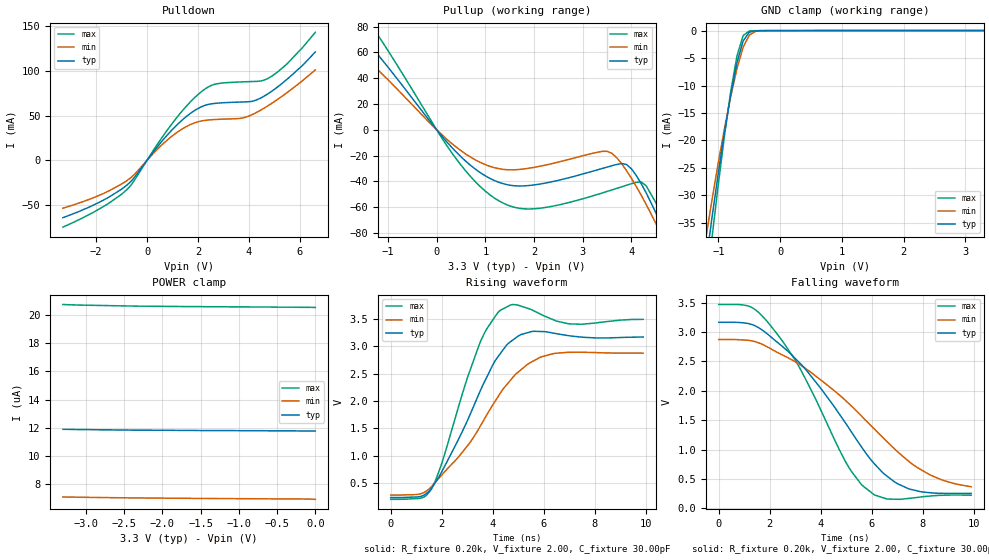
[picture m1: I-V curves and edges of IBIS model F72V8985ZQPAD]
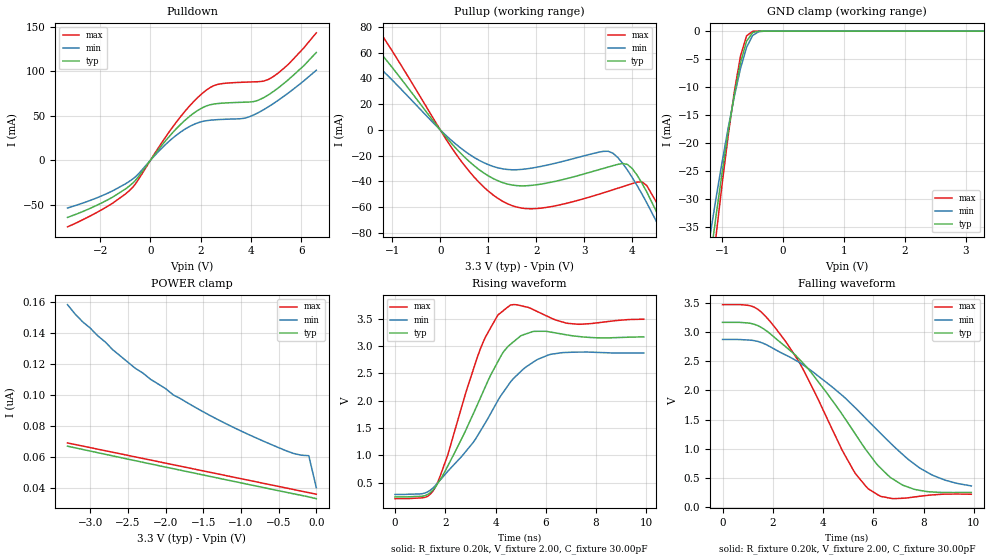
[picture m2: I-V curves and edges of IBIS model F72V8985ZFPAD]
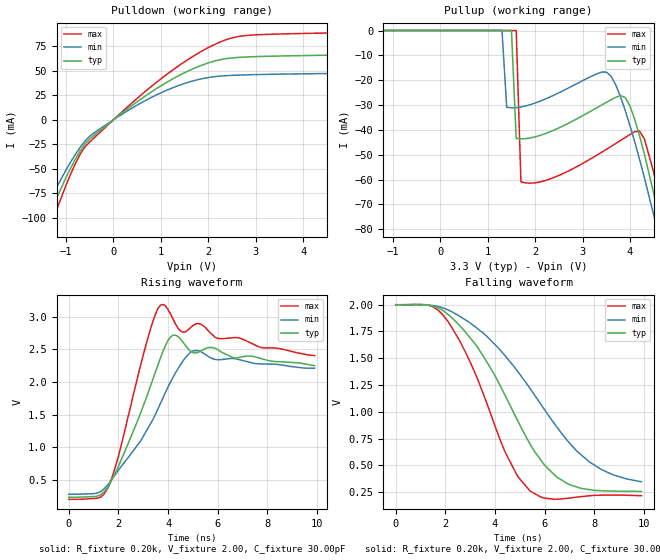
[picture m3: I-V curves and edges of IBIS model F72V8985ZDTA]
| IBIS file f72v8985.ibs created by s2ibis2 version 1.1
| North Carolina State University Electronics Research Laboratory  1995
[IBIS ver]   2.1
[File name]   f72v8985.ibs
[File Rev]   1.0
[Date]   02/03/2000
[Source]   Integrated Device Technology, Inc.
[Notes]   1. Temperatures: typ=25C, min=85C, max=-40C 2. Cemos9_3v
   process. 3. Ramp rates based on 50 ohm load.
[Copyright]   Copyright 1999, Integrated Device Technology, Inc.
|   Component idt72v8985z
[Component]   idt72v8985z
[Manufacturer]   Integrated Device Technology
[Package]
| variable   typ   min   max
R_pkg   0.75   0.60   0.90
L_pkg   8.10nH   8.30nH   9.90nH
C_pkg   0.53pF   0.46pF   0.60pF
[Pin]  signal_name   model_name   R_pin   L_pin   C_pin
1   CCO   F72V8985ZFPAD
2   DTA   F72V8985ZDTA
3   RX0   F72V8985ZTTL
4   RX1   F72V8985ZTTL
5   RX2   F72V8985ZTTL
6   NC   NC
7   RX3   F72V8985ZTTL
8   RX4   F72V8985ZTTL
9   RX5   F72V8985ZTTL
10   RX6   F72V8985ZTTL
11   RX7   F72V8985ZTTL
12   VCC   POWER
13   F0I   F72V8985ZTTL
14   C4I   F72V8985ZTTL
15   A0   F72V8985ZTTL
16   A1   F72V8985ZTTL
17   A2   F72V8985ZTTL
18   NC   NC
19   A3   F72V8985ZTTL
20   A4   F72V8985ZTTL
21   A5   F72V8985ZTTL
22   DS   F72V8985ZTTL
23   R_W   F72V8985ZTTL
24   CS   F72V8985ZTTL
25   D7   F72V8985ZQPAD
26   D6   F72V8985ZQPAD
27   D5   F72V8985ZQPAD
28   NC   NC
29   D4   F72V8985ZQPAD
30   D3   F72V8985ZQPAD
31   D2   F72V8985ZQPAD
32   D1   F72V8985ZQPAD
33   D0   F72V8985ZQPAD
34   GND   GND
35   TX7   F72V8985ZFPAD
36   TX6   F72V8985ZFPAD
37   TX5   F72V8985ZFPAD
38   TX4   F72V8985ZFPAD
39   TX3   F72V8985ZFPAD
40   NC   NC
41   TX2   F72V8985ZFPAD
42   TX1   F72V8985ZFPAD
43   TX0   F72V8985ZFPAD
44   ODE   F72V8985ZTTL
| Models and submodels in the file (4): F72V8985ZQPAD (I/O), F72V8985ZFPAD (3-state), F72V8985ZDTA (Output), F72V8985ZTTL (Input)
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| FIN  FIN   dummy_model
| FOEL FOEL   dummy_model
| QIN  QIN   dummy_model
| QOEL QOEL   dummy_model
| DIN  DIN   dummy_model
|   Model F72V8985ZQPAD
[Model]   F72V8985ZQPAD
Model_type   I/O
Polarity   Non-Inverting
Enable   Active-Low
Vinl =  0.000V
Vinh =  3.000V
Vmeas =  1.500V
C_comp   3.00pF   NA   NA
[Temperature Range]   25.00   85.00   -40.00
[Voltage Range]   3.30V   3.00V   3.60V
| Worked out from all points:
|   slope of the pulldown table from 0 to 0.495 V, typ, clamps not added: 27.2 ohm
|   slope of the pullup table from 0 to 0.495 V, typ, clamps not added: 23.8 ohm
|   GND clamp passes 1 mA (typ) near -0.54 V on its own axis
|   rising waveform, R_fixture 0.20k, V_fixture 2.00, C_fixture 30.00pF: 20-80 % time 1.79ns typ, 2.35ns min, 1.32ns max; typ from 0.239 V to 3.17 V
|   falling waveform, R_fixture 0.20k, V_fixture 2.00, C_fixture 30.00pF: 20-80 % time 3.03ns typ, 3.84ns min, 2.34ns max; typ from 3.17 V to 0.253 V
[Pulldown]
| voltage   I(typ)   I(min)   I(max)
-3.3V     -64.1mA    -53.5mA    -74.7mA
-1.7V     -44.35mA   -36.94mA   -51.5mA
-800mV    -27.94mA   -22.89mA   -33mA
1V        34.54mA    27.43mA    41.66mA
1.6V      50.24mA    38.52mA    62.24mA
2.2V      60.63mA    44.28mA    78.16mA
2.7V      63.7mA     45.63mA    85.25mA
3.8V      65.22mA    47.62mA    87.69mA
4.2V      66.51mA    52.11mA    88.09mA
4.7V      73.5mA     60.13mA    90.8mA
5.5V      90.74mA    75.8mA     108mA
6.6V      121mA      101mA      143mA
[Pullup]
| voltage   I(typ)   I(min)   I(max)
-3.3V     132mA      94.06mA    172mA
-2.3V     105mA      82.04mA    133mA
-1.5V     71.85mA    57.25mA    90.51mA
-1V       48.59mA    38.8mA     61.41mA
400mV     -17.22mA   -13.38mA   -22.49mA
1.4V      -42.19mA   -30.87mA   -57.51mA
2.1V      -42.24mA   -28.46mA   -60.95mA
3.5V      -28.93mA   -16.72mA   -47.84mA
3.9V      -26.98mA   -31.82mA   -43.03mA
4.2V      -41.81mA   -50.76mA   -40.49mA
4.7V      -81.37mA   -88.12mA   -73.82mA
6.6V      -271mA     -258mA     -283mA
[GND_clamp]
| voltage   I(typ)   I(min)   I(max)
-3.3V     -252mA     -218mA     -287mA
-1.2V     -42.01mA   -37.46mA   -47.21mA
-1.1V     -33.66mA   -30.51mA   -37.26mA
-1V       -25.73mA   -23.89mA   -27.78mA
-900mV    -18.33mA   -17.66mA   -18.95mA
-800mV    -11.6mA    -11.94mA   -11.04mA
-700mV    -5.874mA   -6.91mA    -4.622mA
-600mV    -1.891mA   -3.02mA    -905uA
-500mV    -288uA     -824uA     -65.82uA
-400mV    -27.99uA   -134uA     -9.174uA
-300mV    -4.794uA   -17.87uA   -5.389uA
3.3V      11.76uA    6.975uA    20.55uA
[POWER_clamp]
| voltage   I(typ)   I(min)   I(max)
-3.3V     11.88uA    7.058uA    20.77uA
-3.1V     11.86uA    7.04uA     20.73uA
-2.3V     11.82uA    6.987uA    20.65uA
-1.7V     11.8uA     6.961uA    20.62uA
-1.5V     11.79uA    6.954uA    20.62uA
-1.1V     11.79uA    6.94uA     20.6uA
-1V       11.78uA    6.937uA    20.6uA
-700mV    11.78uA    6.928uA    20.59uA
-600mV    11.77uA    6.924uA    20.59uA
-500mV    11.77uA    6.921uA    20.58uA
-100mV    11.76uA    6.911uA    20.57uA
0V        11.76uA    6.889uA    20.56uA
[Ramp]
| variable   typ   min   max
dV/dt_r   1.22/1.36n   0.93/2.27n   1.51/0.86n
dV/dt_f   1.18/3.43n   0.90/4.32n   1.43/2.49n
R_load = 50.00
[Rising Waveform]
R_fixture = 0.20k
V_fixture = 2.00
C_fixture = 30.00pF
R_dut = 0.75
L_dut = 8.10nH
C_dut = 0.53pF
| time   V(typ)   V(min)   V(max)
0s        239mV      284mV      207mV
1.2ns     263mV      311mV      231mV
1.6ns     411mV      442mV      398mV
2ns       712mV      652mV      864mV
3.5ns     2.177V     1.534V     3.067V
4.3ns     2.868V     2.148V     3.656V
5.1ns     3.212V     2.568V     3.731V
6ns       3.266V     2.818V     3.555V
7ns       3.19V      2.888V     3.406V
9.9ns     3.167V     2.872V     3.489V
[Falling Waveform]
R_fixture = 0.20k
V_fixture = 2.00
C_fixture = 30.00pF
R_dut = 0.75
L_dut = 8.10nH
C_dut = 0.53pF
| time   V(typ)   V(min)   V(max)
0s        3.168V     2.875V     3.471V
1.2ns     3.143V     2.859V     3.44V
1.9ns     2.972V     2.75V      3.182V
3.1ns     2.509V     2.473V     2.45V
5.1ns     1.369V     1.784V     699mV
6.1ns     760mV      1.351V     229mV
6.9ns     447mV      1.01V      154mV
7.5ns     326mV      783mV      170mV
8.8ns     254mV      475mV      221mV
9.9ns     253mV      367mV      222mV
|   Model F72V8985ZFPAD
[Model]   F72V8985ZFPAD
Model_type   3-state
Polarity   Non-Inverting
Enable   Active-Low
Vinl =  0.000V
Vinh =  3.000V
Vmeas =  1.500V
C_comp   3.00pF   NA   NA
[Temperature Range]   25.00   85.00   -40.00
[Voltage Range]   3.30V   3.00V   3.60V
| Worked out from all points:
|   slope of the pulldown table from 0 to 0.495 V, typ, clamps not added: 27.1 ohm
|   slope of the pullup table from 0 to 0.495 V, typ, clamps not added: 23.8 ohm
|   GND clamp passes 1 mA (typ) near -0.55 V on its own axis
|   rising waveform, R_fixture 0.20k, V_fixture 2.00, C_fixture 30.00pF: 20-80 % time 1.82ns typ, 2.33ns min, 1.32ns max; typ from 0.239 V to 3.17 V
|   falling waveform, R_fixture 0.20k, V_fixture 2.00, C_fixture 30.00pF: 20-80 % time 3.02ns typ, 3.84ns min, 2.36ns max; typ from 3.17 V to 0.253 V
[Pulldown]
| voltage   I(typ)   I(min)   I(max)
-3.3V     -64.1mA    -53.6mA    -74.7mA
-1.9V     -47.3mA    -39.39mA   -54.9mA
-800mV    -27.95mA   -22.89mA   -33mA
1V        34.55mA    27.44mA    41.67mA
1.6V      50.25mA    38.53mA    62.26mA
2.2V      60.64mA    44.29mA    78.18mA
2.7V      63.71mA    45.64mA    85.27mA
3.8V      65.22mA    47.62mA    87.69mA
4.2V      66.51mA    52.11mA    88.09mA
4.7V      73.5mA     60.13mA    90.8mA
5.5V      90.74mA    75.8mA     108mA
6.6V      121mA      101mA      143mA
[Pullup]
| voltage   I(typ)   I(min)   I(max)
-3.3V     132mA      94.07mA    172mA
-2.3V     105mA      82.05mA    133mA
-1.5V     71.86mA    57.26mA    90.53mA
-1V       48.6mA     38.81mA    61.43mA
400mV     -17.22mA   -13.38mA   -22.49mA
1.4V      -42.19mA   -30.87mA   -57.51mA
2.1V      -42.24mA   -28.46mA   -60.95mA
3.5V      -28.93mA   -16.69mA   -47.84mA
3.9V      -26.91mA   -31.33mA   -43.03mA
4.2V      -41.34mA   -49.81mA   -40.46mA
4.7V      -80.02mA   -86.31mA   -73mA
6.6V      -266mA     -253mA     -278mA
[GND_clamp]
| voltage   I(typ)   I(min)   I(max)
-3.3V     -247mA     -213mA     -281mA
-1.2V     -41.03mA   -36.5mA    -46.2mA
-1.1V     -32.85mA   -29.71mA   -36.43mA
-1V       -25.1mA    -23.25mA   -27.14mA
-900mV    -17.85mA   -17.18mA   -18.49mA
-800mV    -11.28mA   -11.6mA    -10.75mA
-700mV    -5.696mA   -6.698mA   -4.478mA
-600mV    -1.82mA    -2.916mA   -862uA
-500mV    -270uA     -789uA     -54.33uA
-400mV    -22.42uA   -126uA     -1.881uA
-300mV    -1.351uA   -15.02uA   -45.19nA
3.3V      33.1nA     62.2nA     33nA
[POWER_clamp]
| voltage   I(typ)   I(min)   I(max)
-3.3V     66.92nA    158nA      69nA
-3.1V     64.82nA    147nA      67nA
-2.8V     61.7nA     134nA      64nA
-2.7V     60.67nA    129nA      63nA
-2.4V     57.57nA    117nA      60nA
-2V       53.47nA    104nA      56nA
-1.9V     52.45nA    100nA      55nA
-1.3V     46.34nA    83.88nA    49nA
-800mV    41.28nA    72.27nA    44nA
-300mV    36.24nA    62.2nA     39nA
-100mV    34.28nA    60.79nA    37nA
0V        33.12nA    40.23nA    36nA
[Ramp]
| variable   typ   min   max
dV/dt_r   1.22/1.37n   0.93/2.26n   1.51/0.92n
dV/dt_f   1.19/3.43n   0.90/4.32n   1.43/2.49n
R_load = 50.00
[Rising Waveform]
R_fixture = 0.20k
V_fixture = 2.00
C_fixture = 30.00pF
R_dut = 0.75
L_dut = 8.10nH
C_dut = 0.53pF
| time   V(typ)   V(min)   V(max)
0s        239mV      284mV      207mV
1.2ns     263mV      312mV      233mV
1.6ns     415mV      445mV      413mV
2.1ns     806mV      708mV      1.009V
3.4ns     2.053V     1.447V     2.953V
4.1ns     2.72V      2.009V     3.57V
4.5ns     2.994V     2.28V      3.718V
5.4ns     3.252V     2.675V     3.689V
6.2ns     3.255V     2.849V     3.514V
9.9ns     3.167V     2.872V     3.49V
[Falling Waveform]
R_fixture = 0.20k
V_fixture = 2.00
C_fixture = 30.00pF
R_dut = 0.75
L_dut = 8.10nH
C_dut = 0.53pF
| time   V(typ)   V(min)   V(max)
0s        3.168V     2.875V     3.471V
1.2ns     3.142V     2.859V     3.439V
2.1ns     2.898V     2.701V     3.073V
3.4ns     2.378V     2.379V     2.2V
4.8ns     1.566V     1.903V     946mV
5.8ns     931mV      1.478V     315mV
6.3ns     667mV      1.261V     185mV
7.2ns     373mV      892mV      154mV
8.4ns     260mV      541mV      212mV
9.9ns     253mV      365mV      222mV
|   Model F72V8985ZDTA
[Model]   F72V8985ZDTA
Model_type   Output
Vmeas =  1.500V
C_comp   3.00pF   NA   NA
[Temperature Range]   25.00   85.00   -40.00
[Voltage Range]   3.30V   3.00V   3.60V
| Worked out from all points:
|   slope of the pulldown table from 0 to 0.495 V, typ, clamps not added: 27.1 ohm
|   rising waveform, R_fixture 0.20k, V_fixture 2.00, C_fixture 30.00pF: 20-80 % time 1.29ns typ, 1.84ns min, 871ps max; typ from 0.239 V to 2.25 V
|   falling waveform, R_fixture 0.20k, V_fixture 2.00, C_fixture 30.00pF: 20-80 % time 2.53ns typ, 3.29ns min, 1.9ns max; typ from 2 V to 0.256 V
[Pulldown]
| voltage   I(typ)   I(min)   I(max)
-3.3V     -325mA     -279mA     -373mA
-1.7V     -135mA     -115mA     -156mA
-1.5V     -112mA     -95.92mA   -130mA
-900mV    -49.01mA   -42.86mA   -55.09mA
-700mV    -31.48mA   -27.9mA    -34.83mA
-500mV    -19.53mA   -16.73mA   -22.54mA
300mV     11.3mA     9.245mA    13.32mA
1V        34.55mA    27.44mA    41.67mA
1.6V      50.25mA    38.53mA    62.26mA
2.2V      60.64mA    44.29mA    78.18mA
2.9V      64.16mA    45.92mA    86.19mA
6.6V      71.08mA    51.37mA    94.4mA
[Pullup]
| voltage   I(typ)   I(min)   I(max)
-3.3V     66.93nA    151nA      69nA
1.3V      20.08nA    24.27nA    23nA
1.4V      19.08nA    -30.87mA   22nA
1.5V      18.08nA    -31.09mA   21nA
1.6V      -43.45mA   -31.05mA   20nA
1.7V      -43.61mA   -30.78mA   -60.94mA
3.4V      -30mA      -16.74mA   -49.02mA
3.8V      -26.18mA   -26.7mA    -44.24mA
4V        -30.45mA   -38.34mA   -41.84mA
4.3V      -49.54mA   -59.03mA   -43.48mA
4.7V      -83.31mA   -90.44mA   -75.07mA
6.6V      -281mA     -267mA     -293mA
[Ramp]
| variable   typ   min   max
dV/dt_r   0.17/0.28n   0.93/2.28n   1.39/0.80n
dV/dt_f   1.19/3.44n   0.90/4.33n   1.43/2.49n
R_load = 50.00
[Rising Waveform]
R_fixture = 0.20k
V_fixture = 2.00
C_fixture = 30.00pF
R_dut = 0.75
L_dut = 8.10nH
C_dut = 0.53pF
| time   V(typ)   V(min)   V(max)
0s        239mV      284mV      207mV
1.2ns     263mV      312mV      231mV
1.6ns     412mV      443mV      399mV
3.2ns     1.843V     1.303V     2.694V
3.7ns     2.378V     1.682V     3.178V
4.2ns     2.717V     2.075V     2.963V
4.6ns     2.611V     2.324V     2.764V
5ns       2.451V     2.476V     2.866V
5.8ns     2.527V     2.357V     2.719V
9.9ns     2.251V     2.211V     2.406V
[Falling Waveform]
R_fixture = 0.20k
V_fixture = 2.00
C_fixture = 30.00pF
R_dut = 0.75
L_dut = 8.10nH
C_dut = 0.53pF
| time   V(typ)   V(min)   V(max)
0s        2V         2V         2V
1.4ns     1.991V     1.995V     1.991V
2.1ns     1.911V     1.952V     1.845V
3.5ns     1.53V      1.74V      1.186V
4.4ns     1.157V     1.525V     628mV
5.4ns     703mV      1.222V     263mV
6ns       501mV      1.018V     193mV
7ns       319mV      708mV      194mV
8.3ns     262mV      459mV      221mV
9.9ns     256mV      347mV      216mV
